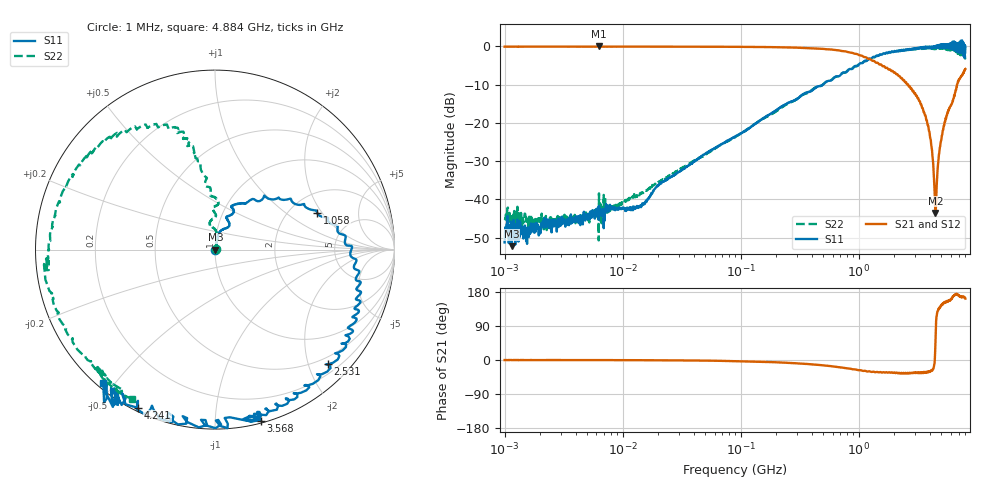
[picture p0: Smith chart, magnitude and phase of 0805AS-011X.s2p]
!s-Parameter Generated by FASTRON Sdn. Bhd.
!FASTRON P/N : 0805AS-011X
!Keysight Technologies: E5071C_MY46733604_B.14.02
!Date: Mon Jun 15 12:48:44 2026
!Version  :Rev01  Mon Jun 15 12:48:44 2026
!Data & Calibration Information:
!Freq  S11:SOLT2(ON)  S21:SOLT2(ON)  S12:SOLT2(ON)  S22:SOLT2(ON)
!PortZ  Port1:50+j0  Port2:50+j0
!When reading reference impedance value at option line is always used.
! Remarks : This data is being provided solely for informational purposes.
# Hz S dB R 50
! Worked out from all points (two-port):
!   1601 points, 1 MHz to 8 GHz, reference 50 ohm
!   highest |S21| = -0.01 dB at 6.301 MHz (marker M1); lowest = -43.5 dB at 4.465 GHz (marker M2)
!   |S21| within 3 dB of the highest: start of sweep to 1.174 GHz
!   lowest |S11| = -52.2 dB at 1.152 MHz (marker M3), VSWR 1.00, Z = 50.2 + j0.0114 ohm
!   |S11| at or under -10 dB: start of sweep to 496.1 MHz
!   |S22| runs from -50.7 to -0.3 dB; largest |S21 - S12| = 0.019
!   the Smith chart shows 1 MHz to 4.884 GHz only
!   S11 on the Smith chart (normalised r, x): 1 MHz: 1.01, -0.00; 1.058 GHz: 2.78, +1.80; 2.531 GHz: 0.36, -2.34; 3.568 GHz: 0.02, -1.31; 4.241 GHz: 0.01, -0.62; 4.884 GHz: 0.02, -0.47
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1000000  -51.20 -2.0  -0.06 -0.1  -0.04 -0.1  -45.40 8.6
1151819  -52.20 2.6  -0.06 -0.1  -0.04 -0.0  -44.40 10.5
4479405  -45.30 30.5  -0.05 -0.2  -0.05 -0.2  -45.20 34.5
6301378  -41.70 38.6  -0.01 -0.4  -0.04 -0.4  -38.40 43.0
1.406113e7  -41.70 67.6  -0.04 -0.5  -0.06 -0.6  -38.30 55.9
2.00676e7  -36.20 66.5  -0.05 -0.7  -0.07 -0.7  -35.50 70.3
8.994653e7  -23.50 78.0  -0.09 -2.9  -0.10 -2.9  -23.70 82.5
4.006501e8  -11.50 68.1  -0.47 -11.6  -0.47 -11.6  -11.40 86.2
1.058419e9  -4.37 19.9  -2.40 -27.9  -2.40 -28.0  -4.43 104.0
1.7949e9  -1.52 -16.0  -6.05 -32.5  -6.05 -32.8  -1.54 128.0
2.530914e9  -0.94 -45.4  -9.56 -35.8  -9.60 -35.9  -1.00 153.0
3.568312e9  -0.11 -74.9  -17.20 -31.3  -17.10 -31.5  -0.39 -175.0
4.014226e9  -0.49 -106.0  -23.70 -30.4  -23.60 -30.8  -0.58 -148.0
4.240668e9  -0.17 -116.0  -29.60 -23.7  -29.60 -23.9  -0.57 -138.0
4.464603e9  0.07 -123.0  -43.50 50.5  -43.60 50.1  -0.52 -133.0
4.632554e9  0.17 -122.0  -33.10 128.0  -33.10 128.0  -0.54 -134.0
4.88448e9  -0.28 -130.0  -26.20 139.0  -26.20 139.0  -0.42 -119.0
5.472309e9  -0.32 -151.0  -18.90 152.0  -18.80 152.0  -0.56 -74.6
5.918038e9  0.77 -153.0  -15.80 159.0  -15.80 158.0  -0.74 -70.1
6.57347e9  -1.09 -169.0  -12.00 172.0  -12.00 172.0  -1.26 -18.9
7.306013e9  1.52 169.0  -7.92 167.0  -7.79 167.0  -1.51 -4.3
8e9  -0.02 135.0  -5.88 162.0  -5.76 161.0  -2.22 32.9
